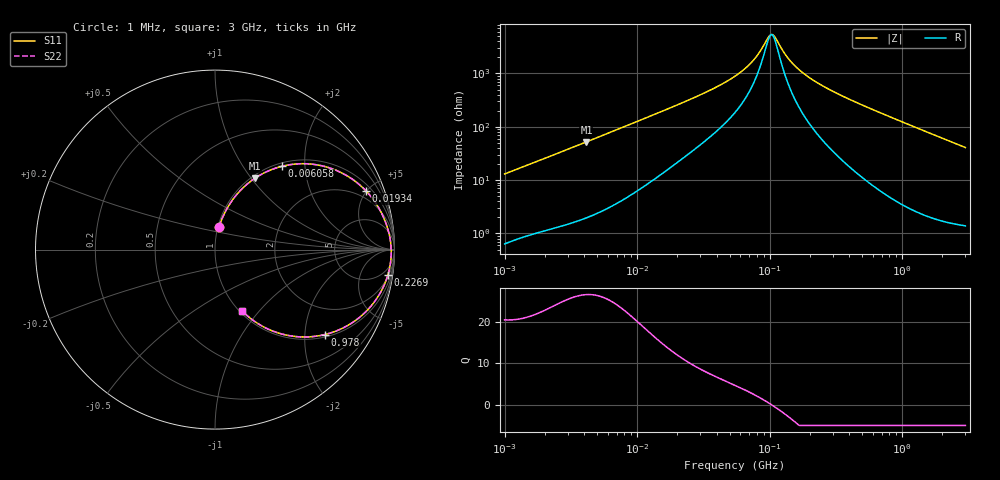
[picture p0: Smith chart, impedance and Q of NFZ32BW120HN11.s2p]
! NFZ32BW120HN11
# Hz S RI R 50
!Freq.(Hz) S11(Real) S11(Imag) S21(Real) S21(Imag) S12(Real) S12(Imag) S22(Real) S22(Imag)
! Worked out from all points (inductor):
!   401 points, 1 MHz to 3 GHz, reference 50 ohm
!   read as one part in series: L = 2.05 uH near 1.041 MHz
!   highest Q = 26.6 at 4.142 MHz (marker M1), where L = 2 uH
!   self-resonance near 103.3 MHz
!   S11 on the Smith chart (normalised r, x): 1 MHz: 1.01, +0.26; 6.058 MHz: 1.06, +1.52; 19.34 MHz: 1.40, +4.93; 226.9 MHz: 2, -13; 978 MHz: 1.07, -2.53; 3 GHz: 1.03, -0.82
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1000000  0.0227 0.1267  0.9773 -0.1267  0.9773 -0.1267  0.0227 0.1267
2182827  0.0807 0.2518  0.9193 -0.2518  0.9193 -0.2518  0.0807 0.2518
3823119  0.1972 0.3794  0.8028 -0.3794  0.8028 -0.3794  0.1972 0.3794
4141799  0.2222 0.3974  0.7778 -0.3974  0.7778 -0.3974  0.2222 0.3974
6058321  0.3718 0.464  0.6282 -0.464  0.6282 -0.464  0.3718 0.464
9223615  0.5705 0.4719  0.4295 -0.4719  0.4295 -0.4719  0.5705 0.4719
1.461624e7  0.7599 0.3959  0.2401 -0.3959  0.2401 -0.3959  0.7599 0.3959
1.934349e7  0.8403 0.3281  0.1597 -0.3281  0.1597 -0.3281  0.8403 0.3281
3.526298e7  0.9355 0.1877  0.0645 -0.1877  0.0645 -0.1877  0.9355 0.1877
5.477226e7  0.9659 0.1039  0.0341 -0.1039  0.0341 -0.1039  0.9659 0.1039
7.395247e7  0.9767 0.0535  0.0233 -0.0535  0.0233 -0.0535  0.9767 0.0535
9.787053e7  0.9814 0.00861  0.0186 -0.00861  0.0186 -0.00861  0.9814 0.00861
1.039275e8  0.9818 -0.00099  0.0182 0.00099  0.0182 0.00099  0.9818 -0.00099
1.103592e8  0.982 -0.0106  0.018 0.0106  0.018 0.0106  0.982 -0.0106
1.460522e8  0.9799 -0.057  0.0201 0.057  0.0201 0.057  0.9799 -0.057
2.094008e8  0.9683 -0.1228  0.0317 0.1228  0.0317 0.1228  0.9683 -0.1228
2.268557e8  0.964 -0.1389  0.036 0.1389  0.036 0.1389  0.964 -0.1389
4.480278e8  0.8813 -0.3002  0.1187 0.3002  0.1187 0.3002  0.8813 -0.3002
8.005644e8  0.7016 -0.4423  0.2984 0.4423  0.2984 0.4423  0.7016 -0.4423
9.779672e8  0.6124 -0.4733  0.3876 0.4733  0.3876 0.4733  0.6124 -0.4733
1.581072e9  0.3797 -0.4723  0.6203 0.4723  0.6203 0.4723  0.3797 -0.4723
3e9  0.1513 -0.3417  0.8487 0.3417  0.8487 0.3417  0.1513 -0.3417
